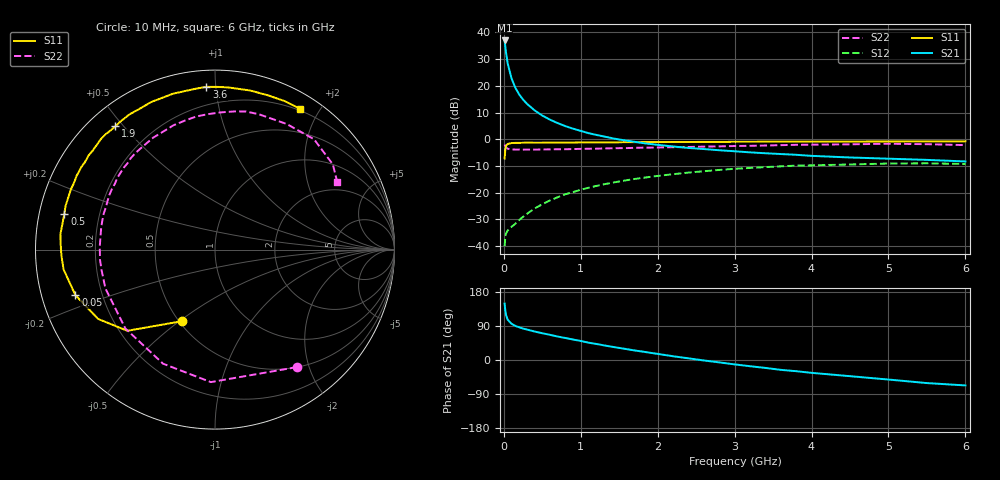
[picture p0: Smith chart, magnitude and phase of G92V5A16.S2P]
! SIEMENS Small Signal Semiconductors
! BFG235
! Si NPN RF Bipolar Junction Transistor in SOT223
! VCE = 2.5 V  IC = 160 mA
! Common Emitter S-Parameters:  July  1994
# GHz  S  MA  R  50
!  f  S11  S21  S12  S22
! GHz  MAG  ANG  MAG  ANG  MAG  ANG  MAG  ANG
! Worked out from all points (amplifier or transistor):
!   40 points, 10 MHz to 6 GHz, reference 50 ohm
!   highest |S21| = 37.0 dB at 10 MHz (marker M1)
!   |S21| within 3 dB of that: start of sweep to 22.21 MHz
!   unconditionally stable (mu >= 1): 435.7 MHz to 1.565 GHz
!   at 200 MHz: K = 0.82, MSG = 23.5 dB, |S12| = -30.2 dB
!   at 1.5 GHz: K = 1.01, MAG = 7.2 dB, |S12| = -15.8 dB
!   at 6 GHz: K = 0.92, MSG = 0.5 dB, |S12| = -9.2 dB
!   S11 on the Smith chart (normalised r, x): 10 MHz: 0.52, -0.51; 50 MHz: 0.10, -0.16; 500 MHz: 0.07, +0.12; 1.9 GHz: 0.08, +0.48; 3.6 GHz: 0.09, +0.94; 6 GHz: 0.18, +1.76
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0.01  0.4379 -114.5  70.77 148.9  0.01 58.5  0.7982 -55.1
0.02  0.6658 -137.2  53.25 129.1  0.0154 43.8  0.7386 -91.8
0.03  0.757 -149.3  40.44 117.8  0.0174 37.8  0.6984 -114.5
0.05  0.818 -161.9  26.32 106.3  0.0196 33.0  0.6652 -138.7
0.1  0.8511 -172.6  13.74 95.5  0.023 36.7  0.6477 -160.5
0.15  0.8563 -177.9  9.193 89.9  0.0264 43.5  0.6422 -169.7
0.2  0.8588 179.4  6.872 86.3  0.0309 48.4  0.6432 -174.8
0.25  0.8622 176.6  5.537 82.9  0.0355 52.1  0.6415 -178.5
0.3  0.8654 174.2  4.622 80.4  0.0403 54.7  0.6423 178.3
0.4  0.8621 170.0  3.482 75.1  0.0507 57.1  0.6419 173.5
0.5  0.8629 166.6  2.783 70.6  0.061 58.3  0.6453 169.5
0.7  0.8679 159.9  2.01 61.9  0.0825 57.4  0.6517 162.2
0.9  0.8693 154.7  1.58 54.0  0.1031 54.2  0.6568 155.9
1.1  0.8753 148.2  1.305 45.8  0.1239 50.5  0.6662 149.6
1.4  0.8765 141.0  1.054 35.1  0.1529 44.2  0.6786 140.9
1.9  0.8831 128.9  0.818 19.1  0.1978 33.1  0.699 126.9
2.2  0.8913 122.3  0.734 9.9  0.2225 26.2  0.7124 118.9
3.2  0.8988 101.0  0.57 -16.4  0.2915 2.9  0.7556 93.0
3.6  0.9083 93.0  0.53 -26.0  0.312 -6.9  0.7769 82.2
4.5  0.9079 77.6  0.457 -42.7  0.3381 -26.2  0.8059 60.2
5.5  0.9143 64.6  0.412 -60.9  0.3551 -47.6  0.8103 35.9
6  0.9166 58.7  0.385 -67.1  0.3453 -55.7  0.7781 28.9
